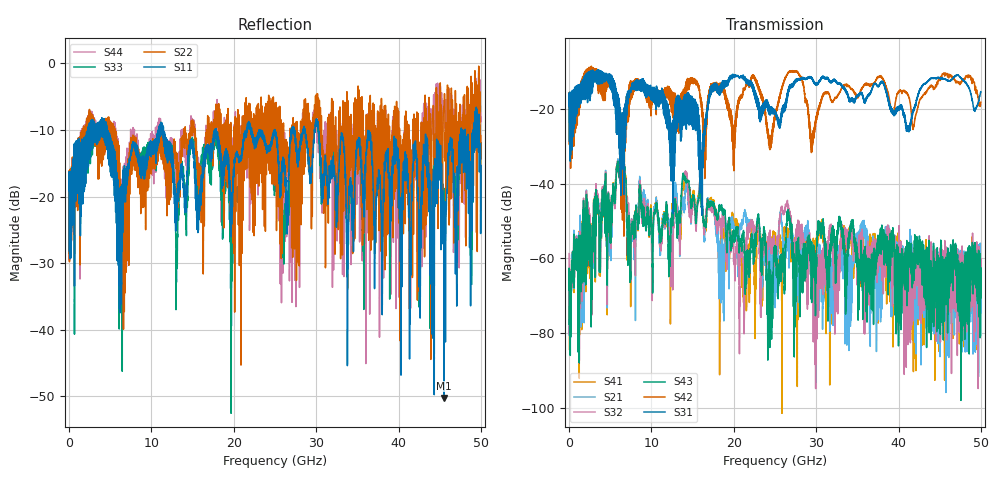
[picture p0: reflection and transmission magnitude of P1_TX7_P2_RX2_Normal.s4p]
!Keysight Technologies,N5225B,MY57041031,A.13.20.10
!Date: Friday, May 31, 2019 11:30:27
!Correction: S11(Full 4 Port(1,2,3,4))
!S12(Full 4 Port(1,2,3,4))
!S13(Full 4 Port(1,2,3,4))
!S14(Full 4 Port(1,2,3,4))
!S21(Full 4 Port(1,2,3,4))
!S22(Full 4 Port(1,2,3,4))
!S23(Full 4 Port(1,2,3,4))
!S24(Full 4 Port(1,2,3,4))
!S31(Full 4 Port(1,2,3,4))
!S32(Full 4 Port(1,2,3,4))
!S33(Full 4 Port(1,2,3,4))
!S34(Full 4 Port(1,2,3,4))
!S41(Full 4 Port(1,2,3,4))
!S42(Full 4 Port(1,2,3,4))
!S43(Full 4 Port(1,2,3,4))
!S44(Full 4 Port(1,2,3,4))
!S4P File: Measurements: <S11,S12,S13,S14>,
!<S21,S22,S23,S24>,
!<S31,S32,S33,S34>,
!<S41,S42,S43,S44>:
# Hz S  dB  R 50.0
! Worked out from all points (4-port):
!   5000 points, 10 MHz to 50 GHz, reference 50 ohm
!   strongest paths, dB at 10 MHz, 12.51 GHz, 25.01 GHz, 37.51 GHz, 50 GHz:
!     S31: -19.4, -38.5, -20.9, -14.0, -15.5
!     S42: -19.4, -15.9, -21.9, -11.5, -18.3
!     S43: -68.4, -47.8, -57.3, -55.0, -66.1
!     S32: -58.7, -54.8, -57.8, -59.9, -64.0
!     S21: -65.7, -48.4, -67.9, -76.3, -64.1
!     S41: -66.7, -45.4, -54.9, -63.1, -61.0
!   lowest |S11| = -50.2 dB at 45.52 GHz (marker M1), VSWR 1.01, Z = 50.2 + j0.19 ohm
!   |S11| at or under -10 dB: 4.613 GHz to 10.86 GHz (6.246 GHz wide, 80.7 % of centre); 11.46 GHz to 17.73 GHz (6.278 GHz wide, 43 % of centre); 30.28 GHz to 47.6 GHz (17.32 GHz wide, 44.5 % of centre)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
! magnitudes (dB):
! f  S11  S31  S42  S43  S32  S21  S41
! 10 MHz  -19.1  -19.4  -19.4  -68.4  -58.7  -65.7  -66.7
! 6.03 GHz  -24.8  -19.6  -18.3  -35.7  -36.1  -35.8  -35.4
! 24.48 GHz  -12.1  -21.4  -29.4  -73.7  -56.1  -60.3  -55.2
! 26.65 GHz  -17.4  -15.3  -10.4  -47.5  -47.3  -55.3  -54.1
! 29.83 GHz  -10.3  -13.4  -24.2  -59.9  -65.6  -67.6  -60.6
! 45.52 GHz  -50.2  -12.0  -10.5  -63.3  -70.1  -61.8  -71.1
! 50 GHz  -15.4  -15.5  -18.3  -66.1  -64.0  -64.1  -61.0
